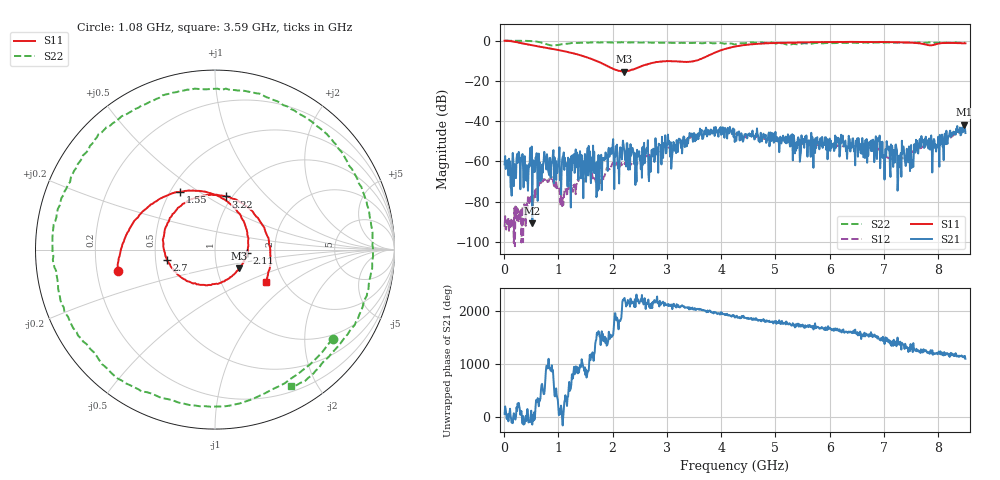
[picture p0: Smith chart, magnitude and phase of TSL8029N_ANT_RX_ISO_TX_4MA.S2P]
!Agilent Technologies,E5071C,MY46523237,B.13.01
!Date: Wed Oct 18 11:02:46 2023
!Data & Calibration Information:
!Freq	S11:SOLT2(ON)	S21:SOLT2(ON)	S12:SOLT2(ON)	S22:SOLT2(ON)
!PortZ  Port1:50+j0  Port2:50+j0
!Above PortZ is port z conversion or system Z0 setting when saving the data.
!When reading, reference impedance value at option line is always used.
# Hz S dB R 50
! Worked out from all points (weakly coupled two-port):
!   850 points, 10 MHz to 8.5 GHz, reference 50 ohm
!   highest |S21| = -41.76 dB at 8.47 GHz (marker M1); lowest = -90.8 dB at 520 MHz (marker M2)
!   lowest |S11| = -15.4 dB at 2.21 GHz (marker M3), VSWR 1.41, Z = 63.7 - j13.7 ohm
!   |S11| at or under -10 dB: 1.694 GHz to 3.522 GHz (1.828 GHz wide, 70.1 % of centre)
!   |S22| runs from -2.4 to 0.1 dB; largest |S21 - S12| = 0.0043
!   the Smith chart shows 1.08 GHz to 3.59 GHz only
!   S11 on the Smith chart (normalised r, x): 1.08 GHz: 0.29, -0.10; 1.55 GHz: 0.56, +0.42; 2.11 GHz: 1.43, -0.06; 2.7 GHz: 0.57, -0.07; 3.22 GHz: 0.94, +0.61; 3.59 GHz: 1.62, -0.66
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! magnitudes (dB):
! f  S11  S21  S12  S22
! 10 MHz  0.0  -61.4  -92.4  0.1
! 520 MHz  -2.3  -90.8  -77.3  -0.3
! 860 MHz  -4.0  -68.0  -68.0  -2.4
! 1.08 GHz  -5.1  -57.7  -78.1  -1.7
! 1.43 GHz  -7.5  -56.8  -65.4  -1.0
! 1.55 GHz  -8.5  -66.9  -64.0  -1.1
! 1.71 GHz  -10.2  -77.0  -69.3  -0.9
! 1.97 GHz  -13.5  -53.4  -62.5  -0.9
! 2.11 GHz  -15.0  -60.8  -62.0  -0.9
! 2.21 GHz  -15.4  -53.6  -60.8  -0.9
! 2.61 GHz  -12.0  -56.3  -57.1  -0.9
! 2.7 GHz  -11.3  -65.2  -57.2  -1.0
! 2.84 GHz  -10.6  -65.6  -56.1  -1.0
! 3.22 GHz  -10.4  -48.7  -50.7  -1.1
! 3.59 GHz  -9.5  -46.0  -46.6  -1.2
! 4.26 GHz  -2.9  -48.0  -46.3  -1.9
! 5.67 GHz  -0.8  -52.8  -51.6  -1.5
! 7.09 GHz  -0.8  -54.5  -58.2  -0.9
! 7.28 GHz  -0.8  -57.1  -59.4  -0.9
! 7.68 GHz  -1.5  -52.8  -53.4  -1.1
! 8.47 GHz  -1.3  -41.8  -44.8  -1.2
! 8.5 GHz  -1.4  -45.9  -44.7  -0.9
